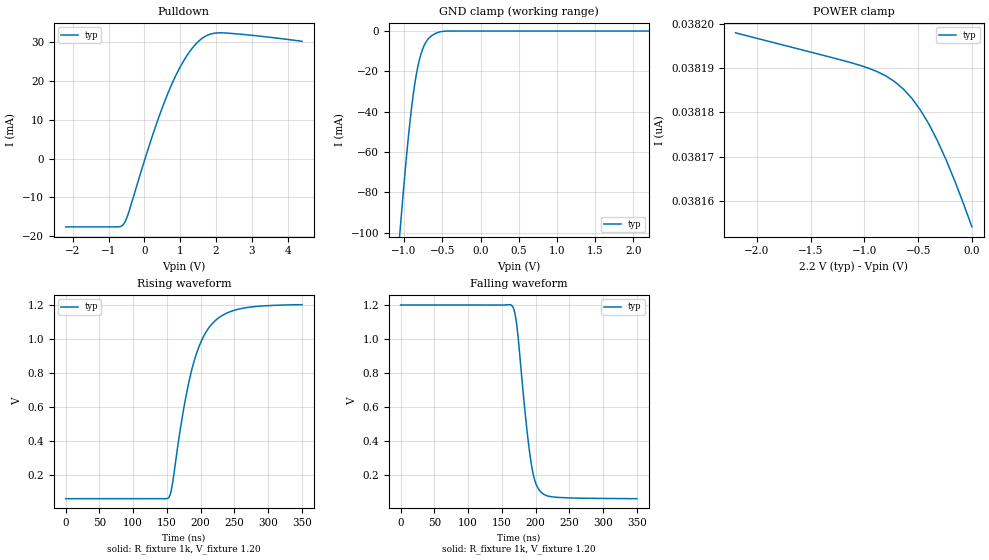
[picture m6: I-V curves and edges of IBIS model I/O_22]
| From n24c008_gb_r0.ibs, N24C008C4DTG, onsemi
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|//////////////////////////////////////////////////////////////////////////////
|//////////////////////////////////////////////////////////////////////////////
[Model] I/O_22
Model_type I/O_open_drain
Vinh =  0.96
Vinl =  0.24
Vmeas = 0.60
Vref = 1.20
Rref = 1000
Cref = 100pF
|  variable   typ   min   max
C_comp   4.60pF   4.60pF   4.60pF
|//////////////////////////////////////////////////////////////////////////////
[Temperature Range]   25   125   -40
|//////////////////////////////////////////////////////////////////////////////
[Voltage Range]   2.20V   2.20V   2.20V
|//////////////////////////////////////////////////////////////////////////////
[Pulldown Reference]   0V   0V   0V
|//////////////////////////////////////////////////////////////////////////////
[POWER Clamp Reference] 2.20V   2.20V   2.20V
|//////////////////////////////////////////////////////////////////////////////
[GND Clamp Reference]   0V   0V   0V
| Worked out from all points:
|   slope of the pulldown table from 0 to 0.33 V, typ, clamps not added: 35.3 ohm
|   GND clamp passes 1 mA (typ) near -0.58 V on its own axis
|   falling waveform, R_fixture 1k, V_fixture 1.20: 20-80 % time 17.7ns typ, NA min, NA max; typ from 1.2 V to 0.06 V
|   rising waveform, R_fixture 1k, V_fixture 1.20: 20-80 % time 36.2ns typ, NA min, NA max; typ from 0.06 V to 1.2 V
|//////////////////////////////////////////////////////////////////////////////
[Pulldown]
|   Voltage   I(typ)   I(min)   I(max)
-2.2V     -17.63mA   NA         NA
-740mV    -17.63mA   NA         NA
-560mV    -16.62mA   NA         NA
-440mV    -13.92mA   NA         NA
280mV     7.424mA    NA         NA
680mV     17.37mA    NA         NA
920mV     22.23mA    NA         NA
1.16V     26.18mA    NA         NA
1.58V     30.79mA    NA         NA
1.82V     32.04mA    NA         NA
2.18V     32.43mA    NA         NA
4.4V      30.25mA    NA         NA
|//////////////////////////////////////////////////////////////////////////////
[GND Clamp]
|   Voltage   I(typ)   I(min)   I(max)
-2.2V     -618.5mA   NA         NA
-1.08V    -111.3mA   NA         NA
-1.04V    -93.22mA   NA         NA
-980mV    -66.89mA   NA         NA
-940mV    -51.12mA   NA         NA
-880mV    -31.47mA   NA         NA
-840mV    -21.58mA   NA         NA
-800mV    -14.31mA   NA         NA
-740mV    -7.368mA   NA         NA
-620mV    -1.831mA   NA         NA
-420mV    -16.46uA   NA         NA
2.2V      38.15nA    NA         NA
|//////////////////////////////////////////////////////////////////////////////
[POWER Clamp]
|   Voltage   I(typ)   I(min)   I(max)
-2.2V     38.2nA     NA         NA
-1.04V    38.19nA    NA         NA
-880mV    38.19nA    NA         NA
-720mV    38.19nA    NA         NA
-640mV    38.19nA    NA         NA
-560mV    38.18nA    NA         NA
-480mV    38.18nA    NA         NA
-400mV    38.18nA    NA         NA
-320mV    38.17nA    NA         NA
-240mV    38.17nA    NA         NA
-160mV    38.16nA    NA         NA
0V        38.15nA    NA         NA
|//////////////////////////////////////////////////////////////////////////////
|//////////////////////////////////////////////////////////////////////////////
[Ramp]
|  variable   typ   min   max
dV/dt_r   1.265E-00/2.500E-10  NA   NA
dV/dt_f   1.265E-00/1.800E-08  NA   NA
R_load = 1k
|//////////////////////////////////////////////////////////////////////////////
|//////////////////////////////////////////////////////////////////////////////
[Falling Waveform]
R_fixture = 1k
V_fixture = 1.20
V_fixture_min = 1.10
V_fixture_max = 1.30
C_fixture = 0p
|   time   V(typ)   V(min)   V(max)
0s        1.2V       NA         NA
164ns     1.199V     NA         NA
168ns     1.171V     NA         NA
172ns     1.081V     NA         NA
185ns     541.6mV    NA         NA
193ns     278.2mV    NA         NA
198ns     177.4mV    NA         NA
204ns     118.4mV    NA         NA
228ns     69.2mV     NA         NA
350ns     60mV       NA         NA
|//////////////////////////////////////////////////////////////////////////////
[Rising Waveform]
R_fixture = 1k
V_fixture = 1.20
V_fixture_min = 1.10
V_fixture_max = 1.30
C_fixture = 0p
|   time   V(typ)   V(min)   V(max)
0s        60mV       NA         NA
151.5ns   62.52mV    NA         NA
157.5ns   131.5mV    NA         NA
172.5ns   534.8mV    NA         NA
184.5ns   780.6mV    NA         NA
196.5ns   943.2mV    NA         NA
210ns     1.053V     NA         NA
227.5ns   1.125V     NA         NA
255ns     1.173V     NA         NA
350ns     1.2V       NA         NA
